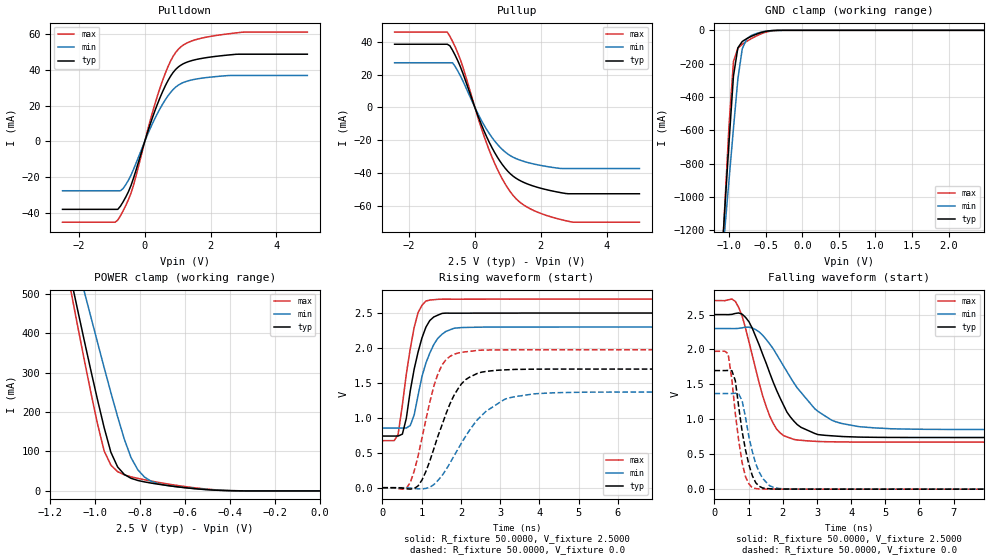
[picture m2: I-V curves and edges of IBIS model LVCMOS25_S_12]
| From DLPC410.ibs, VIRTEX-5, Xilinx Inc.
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|   Model LVCMOS25_S_12
[Model]  LVCMOS25_S_12
Model_type I/O
Polarity   Non-Inverting
Enable   Active-Low
Vinl = 0.65
Vinh = 1.85
Vmeas =  1.2500V
Cref =   0.0F
Rref =   1.0000M
Vref =   0.0V
C_comp   6.0000pF   6.0000pF   6.0000pF
[Model Spec]
Vinl   0.65   0.6   0.7
Vinh   1.85   1.7   2.0
[Temperature Range]   25.0000   85.0000   0.0
[Voltage Range]   2.5000V   2.3000V   2.7000V
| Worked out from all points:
|   slope of the pulldown table from 0 to 0.375 V, typ, clamps not added: 18.3 ohm
|   slope of the pullup table from 0 to 0.375 V, typ, clamps not added: 20 ohm
|   GND clamp passes 1 mA (typ) near -0.39 V on its own axis
|   POWER clamp passes 1 mA (typ) near -0.43 V on its own axis
|   rising waveform, R_fixture 50.0000, V_fixture 2.5000: 20-80 % time 376ps typ, 432ps min, 328ps max; typ from 0.74 V to 2.5 V
|   rising waveform, R_fixture 50.0000, V_fixture 0.0: 20-80 % time 684ps typ, 1.01ns min, 503ps max; typ from 0 V to 1.7 V
|   falling waveform, R_fixture 50.0000, V_fixture 2.5000: 20-80 % time 900ps typ, 1.24ns min, 679ps max; typ from 2.5 V to 0.74 V
|   falling waveform, R_fixture 50.0000, V_fixture 0.0: 20-80 % time 352ps typ, 404ps min, 298ps max; typ from 1.7 V to 0 V
[Pulldown]
|Voltage   I(typ)   I(min)   I(max)
-2.5V     -38.19mA   -27.75mA   -45.4mA
-900mV    -38.19mA   -27.75mA   -45.4mA
-820mV    -38.19mA   -27.75mA   -44.17mA
-660mV    -34.01mA   -26.53mA   -39.08mA
-420mV    -24.85mA   -19.05mA   -29.15mA
140mV     8.212mA    6.157mA    9.988mA
540mV     27.82mA    20.82mA    34.08mA
860mV     38.62mA    29.04mA    47.66mA
1.1V      42.79mA    32.41mA    53.07mA
1.66V     46.29mA    35.24mA    57.61mA
2.7V      48.72mA    36.96mA    60.69mA
4.94V     48.9mA     36.96mA    61.3mA
[Pullup]
|Voltage   I(typ)   I(min)   I(max)
-2.44V    38.57mA    27.27mA    45.99mA
-840mV    38.57mA    27.27mA    45.99mA
-680mV    34.91mA    27.27mA    40.36mA
-600mV    31.85mA    24.98mA    36.97mA
-360mV    20.56mA    15.97mA    24.36mA
200mV     -10.61mA   -8.007mA   -12.92mA
600mV     -27.55mA   -20.5mA    -34.11mA
1V        -38.97mA   -28.46mA   -49.3mA
1.4V      -44.98mA   -32.4mA    -58.39mA
2.04V     -49.56mA   -35.57mA   -65.02mA
2.92V     -52.73mA   -37.31mA   -69.88mA
5V        -52.73mA   -37.31mA   -70.08mA
[GND_clamp]
|Voltage   I(typ)   I(min)   I(max)
-2.5V     -11.3A     -8.702A    -13.55A
-1.12V    -1.504A    -1.514A    -1.577A
-1.06V    -1.082A    -1.202A    -1.064A
-1V       -666.6mA   -893.1mA   -565.5mA
-940mV    -273.3mA   -587.1mA   -186.2mA
-880mV    -105.1mA   -292.6mA   -107.5mA
-820mV    -66.91mA   -110.8mA   -83.73mA
-760mV    -50.05mA   -51.73mA   -66.37mA
-700mV    -36.88mA   -31.85mA   -50.72mA
-520mV    -8.293mA   -6.886mA   -14.09mA
-340mV    -253.5uA   -293.6uA   -653.8uA
2.48V     378.6nA    5.297uA    366.7nA
[POWER_clamp]
|Voltage   I(typ)   I(min)   I(max)
-2.49V    4.212A     3.665A     4.661A
-1.11V    543.2mA    639.6mA    512.7mA
-1.08V    463.8mA    573.9mA    423.6mA
-1.05V    384.8mA    508.3mA    336.3mA
-1.02V    307.4mA    442.8mA    251.7mA
-960mV    160.5mA    312.5mA    101.5mA
-930mV    98.04mA    249.2mA    65.3mA
-900mV    60.83mA    188.2mA    48.87mA
-840mV    31.95mA    84.25mA    35.72mA
-780mV    22.84mA    35.01mA    28.28mA
-540mV    4.801mA    5.183mA    6.815mA
0V        384.3nA    408.9nA    427.5nA
[Ramp]
dV/dt_r  1.0188/0.6744n   0.8214/0.9981n   1.1844/0.5028n
dV/dt_f  1.0563/0.8905n   0.8677/1.2284n   1.2158/0.6687n
R_load = 50.0000
[Rising Waveform]
R_fixture= 50.0000
V_fixture= 2.5000
V_fixture_min= 2.3000
V_fixture_max= 2.7000
|time   V(typ)   V(min)   V(max)
0s        739.5mV    853.9mV    673.7mV
400ps     739.3mV    853.9mV    759.3mV
510ps     766.8mV    853.9mV    1.184V
710ps     1.384V     889.4mV    1.986V
810ps     1.697V     1.041V     2.294V
910ps     1.942V     1.323V     2.507V
1.11ns    2.299V     1.786V     2.672V
1.41ns    2.469V     2.136V     2.696V
1.92ns    2.498V     2.288V     2.698V
10ns      2.5V       2.3V       2.7V
[Rising Waveform]
R_fixture= 50.0000
V_fixture= 0.0
|time   V(typ)   V(min)   V(max)
0s        3.489uV    4.276uV    3.426uV
510ps     -5.746mV   22.11uV    -20.97mV
710ps     -20.08mV   -4.762mV   72.84mV
1.01ns    110.9mV    -16.69mV   712.1mV
1.41ns    729.5mV    100.7mV    1.621V
1.82ns    1.317V     448.2mV    1.909V
2.12ns    1.546V     736.1mV    1.945V
2.42ns    1.636V     972.1mV    1.965V
3.33ns    1.692V     1.298V     1.974V
10ns      1.698V     1.369V     1.974V
[Falling Waveform]
R_fixture= 50.0000
V_fixture= 2.5000
V_fixture_min= 2.3000
V_fixture_max= 2.7000
|time   V(typ)   V(min)   V(max)
0s        2.5V       2.3V       2.7V
510ps     2.503V     2.299V     2.722V
710ps     2.523V     2.303V     2.602V
1.01ns    2.397V     2.319V     2.11V
1.52ns    1.795V     2.141V     1.176V
2.02ns    1.205V     1.765V     766.9mV
2.53ns    885.9mV    1.388V     699.9mV
3.03ns    781.4mV    1.114V     682.9mV
3.74ns    753.7mV    939.1mV    676.1mV
10ns      739.5mV    853.9mV    673.7mV
[Falling Waveform]
R_fixture= 50.0000
V_fixture= 0.0
|time   V(typ)   V(min)   V(max)
0s        1.698V     1.369V     1.974V
400ps     1.7V       1.369V     1.94V
510ps     1.696V     1.369V     1.57V
610ps     1.555V     1.374V     1.084V
810ps     827.2mV    1.267V     380.7mV
910ps     558.4mV    1.026V     175.3mV
1.11ns    190.7mV    535.2mV    18.29mV
1.41ns    16.82mV    154.8mV    2.335mV
1.92ns    1.172mV    8.01mV     885.2uV
10ns      10.42uV    14.49uV    -2.916uV
